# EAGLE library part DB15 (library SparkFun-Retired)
DB15 / VGA right angle through-hole female connector.
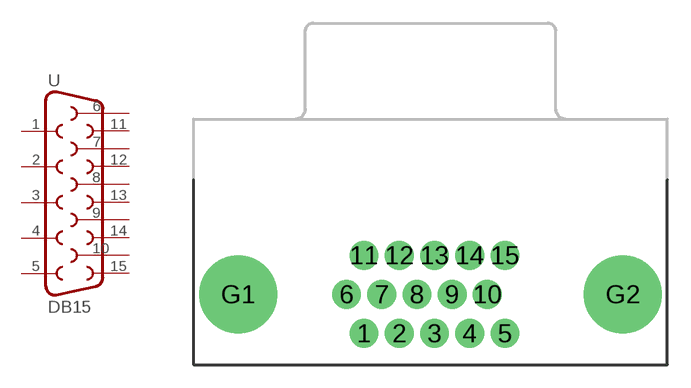
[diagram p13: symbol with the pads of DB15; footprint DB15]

Designator prefix -

## DB15  [DB15]
1  1  pas
2  2  pas
3  3  pas
4  4  pas
5  5  pas
6  6  pas
7  7  pas
8  8  pas
9  9  pas
10  10  pas
11  11  pas
12  12  pas
13  13  pas
14  14  pas
15  15  pas

## Footprint DB15 (pad centres in mm)
drill 1.016 pad 1.88: 1 -4.32,-7.62; 2 -2.03,-7.62; 3 0.26,-7.62; 4 2.55,-7.62; 5 4.84,-7.62; 6 -5.46,-5.08; 7 -3.17,-5.08; 8 -0.88,-5.08; 9 1.41,-5.08; 10 3.7,-5.08; 11 -4.32,-2.54; 12 -2.03,-2.54; 13 0.26,-2.54; 14 2.55,-2.54; 15 4.84,-2.54
drill 3.302 pad 5.08: G1 -12.5,-5.08; G2 12.5,-5.08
